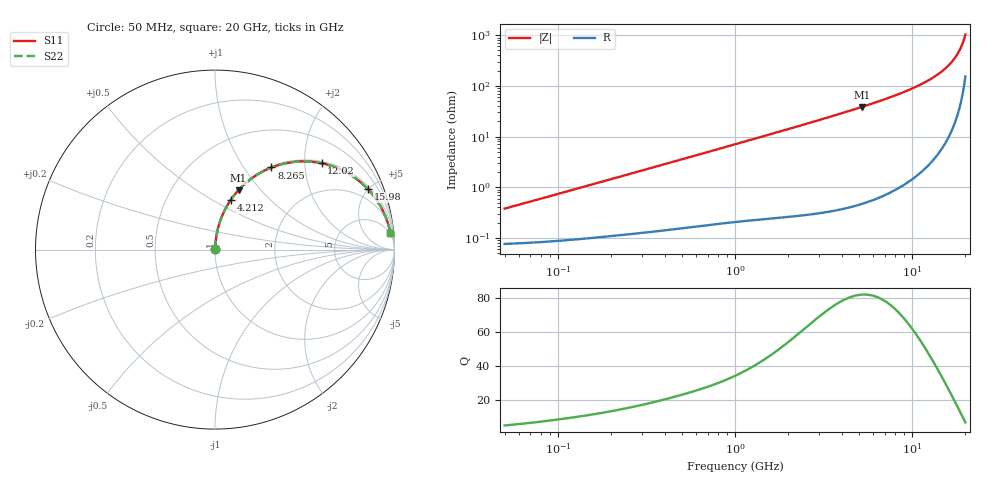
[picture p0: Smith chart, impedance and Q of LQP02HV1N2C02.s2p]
!Murata Part Number: LQP02HV1N2C02
!These Parameters are Measured in Series Mode Connection
!  o--[Z]--o
!Port1  Port2
!  o-------o
!Freq. Start=50[MHz] Stop=20[GHz], 401[Steps]
# Hz S RI R 50
!Freq.(Hz) S11(Real) S11(Imag) S21(Real) S21(Imag) S12(Real) S12(Imag) S22(Real) S22(Imag)
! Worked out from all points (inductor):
!   401 points, 50 MHz to 20 GHz, reference 50 ohm
!   read as one part in series: L = 1.18 nH near 51.52 MHz
!   highest Q = 82 at 5.195 GHz (marker M1), where L = 1.17 nH
!   S11 on the Smith chart (normalised r, x): 50 MHz: 1.00, +0.01; 4.212 GHz: 1.01, +0.61; 8.265 GHz: 1.02, +1.35; 12.02 GHz: 1.05, +2.43; 15.98 GHz: 1.19, +4.96; 20 GHz: 4, +20
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5e7  0.000775 0.00371  0.9992 -0.00371  0.9992 -0.00371  0.000775 0.00371
1.364002e8  0.00106 0.00991  0.9989 -0.00991  0.9989 -0.00991  0.00106 0.00991
3.721004e8  0.00207 0.0264  0.9979 -0.0264  0.9979 -0.0264  0.00207 0.0264
1e9  0.00694 0.0696  0.9931 -0.0696  0.9931 -0.0696  0.00694 0.0696
1.714689e9  0.0166 0.118  0.9834 -0.118  0.9834 -0.118  0.0166 0.118
2.728004e9  0.0385 0.1849  0.9615 -0.1849  0.9615 -0.1849  0.0385 0.1849
4.212059e9  0.0877 0.2766  0.9123 -0.2766  0.9123 -0.2766  0.0877 0.2766
5.194772e9  0.1311 0.3314  0.8689 -0.3314  0.8689 -0.3314  0.1311 0.3314
6.311513e9  0.1901 0.3862  0.8099 -0.3862  0.8099 -0.3862  0.1901 0.3862
7.442007e9  0.2592 0.4317  0.7408 -0.4317  0.7408 -0.4317  0.2592 0.4317
8.264682e9  0.3145 0.4574  0.6855 -0.4574  0.6855 -0.4574  0.3145 0.4574
1.019291e10  0.4555 0.4899  0.5445 -0.4899  0.5445 -0.4899  0.4555 0.4899
1.201863e10  0.5941 0.4811  0.4059 -0.4811  0.4059 -0.4811  0.5941 0.4811
1.314879e10  0.6767 0.4561  0.3233 -0.4561  0.3233 -0.4561  0.6767 0.4561
1.417136e10  0.7463 0.4217  0.2537 -0.4217  0.2537 -0.4217  0.7463 0.4217
1.504638e10  0.8004 0.3843  0.1996 -0.3843  0.1996 -0.3843  0.8004 0.3843
1.597544e10  0.8511 0.3377  0.1489 -0.3377  0.1489 -0.3377  0.8511 0.3377
1.696185e10  0.8964 0.2823  0.1036 -0.2823  0.1036 -0.2823  0.8964 0.2823
1.800918e10  0.9343 0.2187  0.0657 -0.2187  0.0657 -0.2187  0.9343 0.2187
1.88369e10  0.9567 0.1664  0.0433 -0.1664  0.0433 -0.1664  0.9567 0.1664
1.970266e10  0.9731 0.1111  0.0269 -0.1111  0.0269 -0.1111  0.9731 0.1111
2e10  0.9771 0.0922  0.0229 -0.0922  0.0229 -0.0922  0.9771 0.0922
